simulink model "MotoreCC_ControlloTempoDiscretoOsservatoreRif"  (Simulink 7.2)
settings: Solver=ode45  StartTime=0.0  StopTime=10.0  RelTol=1e-3
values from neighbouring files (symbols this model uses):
  A = [0   1   0    [Esercitazione06.m]
  as1 = 2    [Esercitazione06.m]
  as2 = -3    [Esercitazione06.m]
  B = [0  0   1]'    [Esercitazione06.m]
  C = [1  0   0]    [Esercitazione06.m]
  Kcontr = -acker(Az,Bz,[0.9 0 0])    [Esercitazione06.m]
  Kff = -inv(Cz*inv(Az+Bz*Kcontr-eye(m))*Bz)    [Esercitazione06.m]
  L = -acker(Az',Cz',[0 0 0])'    [Esercitazione06.m]
  Ts = 0.1    [Esercitazione06.m]
  ts1 = 2    [Esercitazione06.m]
  ts2 = 10    [Esercitazione06.m]
  X0 = [0.5 2 0.3]'    [Esercitazione06.m]
undefined symbols (not defined in the file or in its folder): Az, Bz, Cz
libraries: simulink x1

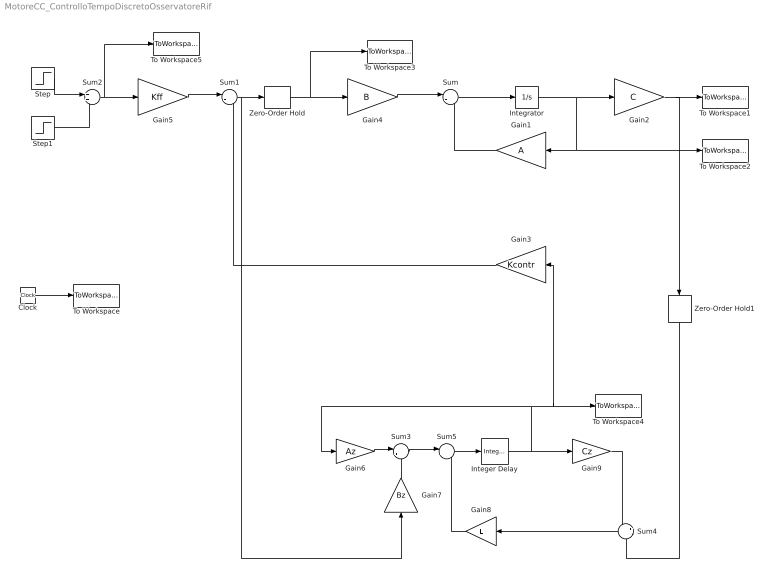
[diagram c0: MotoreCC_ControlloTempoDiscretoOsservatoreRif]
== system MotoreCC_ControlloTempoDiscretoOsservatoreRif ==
  Clock : Clock
  Gain1 : Gain  Orientation=left  Gain=A  Multiplication=Matrix(K*u)  ParameterDataType=sfix(16)  ParameterScaling=2^0  OutDataType=sfix(16)  OutScaling=2^0
  Gain2 : Gain  Gain=C  Multiplication=Matrix(K*u)  ParameterDataType=sfix(16)  ParameterScaling=2^0  OutDataType=sfix(16)  OutScaling=2^0
  Gain3 : Gain  Orientation=left  Gain=Kcontr  Multiplication=Matrix(K*u)  ParameterDataType=sfix(16)  ParameterScaling=2^0  OutDataType=sfix(16)  OutScaling=2^0
  Gain4 : Gain  Gain=B  Multiplication=Matrix(K*u)  ParameterDataType=sfix(16)  ParameterScaling=2^0  OutDataType=sfix(16)  OutScaling=2^0
  Gain5 : Gain  Gain=Kff  Multiplication=Matrix(K*u)  ParameterDataType=sfix(16)  ParameterScaling=2^0  OutDataType=sfix(16)  OutScaling=2^0
  Gain6 : Gain  Gain=Az  Multiplication=Matrix(K*u)  ParameterDataType=sfix(16)  ParameterScaling=2^0  OutDataType=sfix(16)  OutScaling=2^0
  Gain7 : Gain  Orientation=up  Gain=Bz  Multiplication=Matrix(K*u)  ParameterDataType=sfix(16)  ParameterScaling=2^0  OutDataType=sfix(16)  OutScaling=2^0
  Gain8 : Gain  Orientation=left  Gain=L  Multiplication=Matrix(K*u)  ParameterDataType=sfix(16)  ParameterScaling=2^0  OutDataType=sfix(16)  OutScaling=2^0
  Gain9 : Gain  Gain=Cz  Multiplication=Matrix(K*u)  ParameterDataType=sfix(16)  ParameterScaling=2^0  OutDataType=sfix(16)  OutScaling=2^0
  Integer Delay : simulink/Discrete/Integer Delay  vinit=[0 0 0]'  samptime=Ts  NumDelays=1
  Integrator : Integrator  InitialCondition=X0
  Step : Step  Time=ts1  After=as1  SampleTime=0
  Step1 : Step  Time=ts2  After=as2  SampleTime=0
  Sum{,1,3,5} (4 alike) : Sum  Inputs=|++  OutDataType=sfix(16)  OutScaling=2^0
  Sum2 : Sum  OutDataType=sfix(16)  OutScaling=2^0
  Sum4 : Sum  Orientation=left  Inputs=+-  OutDataType=sfix(16)  OutScaling=2^0
  To Workspace : ToWorkspace  VariableName=time  SampleTime=-1  SaveFormat=Array
  To Workspace1 : ToWorkspace  VariableName=y  SampleTime=-1  SaveFormat=Array
  To Workspace2 : ToWorkspace  VariableName=X  SampleTime=-1  SaveFormat=Array
  To Workspace3 : ToWorkspace  VariableName=ud  SampleTime=-1  SaveFormat=Array
  To Workspace4 : ToWorkspace  VariableName=Xs  SampleTime=-1  SaveFormat=Array
  To Workspace5 : ToWorkspace  VariableName=yref  SampleTime=-1  SaveFormat=Array
  Zero-Order Hold : ZeroOrderHold  SampleTime=Ts
  Zero-Order Hold1 : ZeroOrderHold  Orientation=down  SampleTime=Ts
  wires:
  Gain1/1 -> Sum/2
  Sum/1 -> Integrator/1
  Integrator/1 -> Gain2/1, Gain1/1, To Workspace2/1
  Gain2/1 -> To Workspace1/1, Zero-Order Hold1/1
  Gain4/1 -> Sum/1
  Gain3/1 -> Sum1/2
  Clock/1 -> To Workspace/1
  Gain6/1 -> Sum3/1
  Integer Delay/1 -> Gain9/1, Gain6/1, Gain3/1, To Workspace4/1
  Gain7/1 -> Sum3/2
  Sum4/1 -> Gain8/1
  Gain9/1 -> Sum4/1
  Gain8/1 -> Sum5/2
  Sum3/1 -> Sum5/1
  Sum5/1 -> Integer Delay/1
  Zero-Order Hold1/1 -> Sum4/2
  Zero-Order Hold/1 -> Gain4/1, To Workspace3/1
  Sum1/1 -> Zero-Order Hold/1, Gain7/1
  Step/1 -> Sum2/1
  Step1/1 -> Sum2/2
  Sum2/1 -> To Workspace5/1, Gain5/1
  Gain5/1 -> Sum1/1
